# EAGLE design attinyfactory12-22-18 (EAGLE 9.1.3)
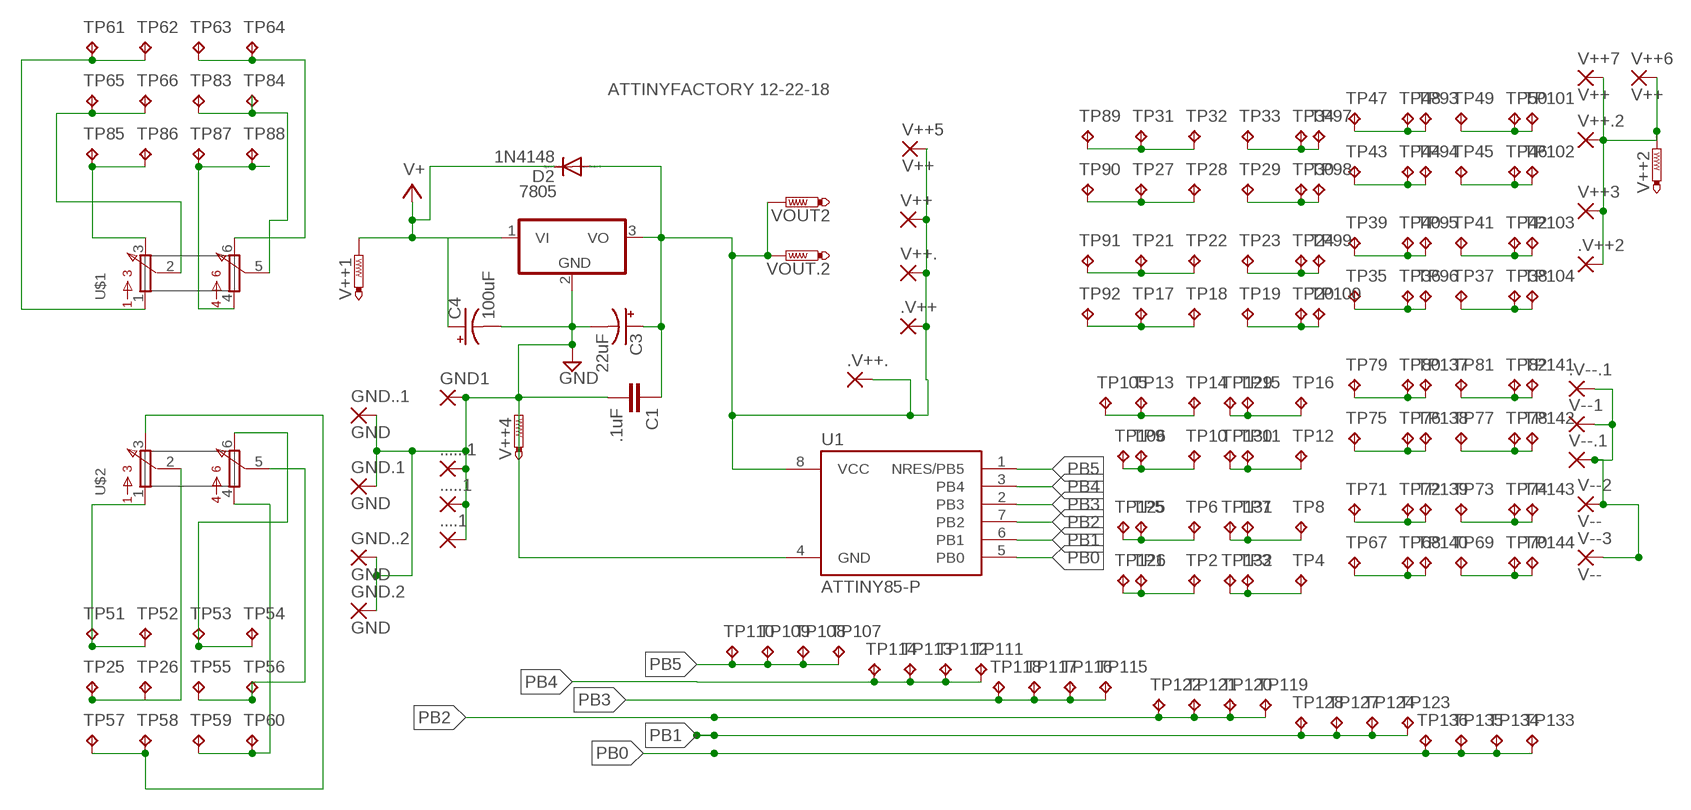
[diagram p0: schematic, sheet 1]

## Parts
7805  7805T  [TO220H]
....1  2,54/0,9  [2,54/0,9]
.....1  2,54/0,9  [2,54/0,9]
......1  2,54/0,9  [2,54/0,9]
.V++  2,54/1,0  [2,54/1,0]
.V++2  2,54/1,0  [2,54/1,0]
.V++.  2,54/1,0  [2,54/1,0]
.V--.1  3,17/1,3  [3,17/1,3]
C1  .1uF  C5/2.5  [C5B2.5]
C3  22uF  CPOL-USE3.5-10  [E3,5-10]
C4  100uF  CPOL-USE3.5-10  [E3,5-10]
D2  1N4148  1N4004  [DO41-10]
GND1  2,54/0,9  [2,54/0,9]
GND.1  GND  1,6/0,8  [1,6/0,8]
GND.2  GND  1,6/0,8  [1,6/0,8]
GND..1  GND  1,6/0,8  [1,6/0,8]
GND..2  GND  1,6/0,8  [1,6/0,8]
TP1  TPPAD1-13  [P1-13]
TP2  TPPAD1-13  [P1-13]
TP3  TPPAD1-13  [P1-13]
TP4  TPPAD1-13  [P1-13]
TP5  TPPAD1-13  [P1-13]
TP6  TPPAD1-13  [P1-13]
TP7  TPPAD1-13  [P1-13]
TP8  TPPAD1-13  [P1-13]
TP9  TPPAD1-13  [P1-13]
TP10  TPPAD1-13  [P1-13]
TP11  TPPAD1-13  [P1-13]
TP12  TPPAD1-13  [P1-13]
TP13  TPPAD1-13  [P1-13]
TP14  TPPAD1-13  [P1-13]
TP15  TPPAD1-13  [P1-13]
TP16  TPPAD1-13  [P1-13]
TP17  TPPAD1-13  [P1-13]
TP18  TPPAD1-13  [P1-13]
TP19  TPPAD1-13  [P1-13]
TP20  TPPAD1-13  [P1-13]
TP21  TPPAD1-13  [P1-13]
TP22  TPPAD1-13  [P1-13]
TP23  TPPAD1-13  [P1-13]
TP24  TPPAD1-13  [P1-13]
TP25  TPPAD1-13  [P1-13]
TP26  TPPAD1-13  [P1-13]
TP27  TPPAD1-13  [P1-13]
TP28  TPPAD1-13  [P1-13]
TP29  TPPAD1-13  [P1-13]
TP30  TPPAD1-13  [P1-13]
TP31  TPPAD1-13  [P1-13]
TP32  TPPAD1-13  [P1-13]
TP33  TPPAD1-13  [P1-13]
TP34  TPPAD1-13  [P1-13]
TP35  TPPAD1-13  [P1-13]
TP36  TPPAD1-13  [P1-13]
TP37  TPPAD1-13  [P1-13]
TP38  TPPAD1-13  [P1-13]
TP39  TPPAD1-13  [P1-13]
TP40  TPPAD1-13  [P1-13]
TP41  TPPAD1-13  [P1-13]
TP42  TPPAD1-13  [P1-13]
TP43  TPPAD1-13  [P1-13]
TP44  TPPAD1-13  [P1-13]
TP45  TPPAD1-13  [P1-13]
TP46  TPPAD1-13  [P1-13]
TP47  TPPAD1-13  [P1-13]
TP48  TPPAD1-13  [P1-13]
TP49  TPPAD1-13  [P1-13]
TP50  TPPAD1-13  [P1-13]
TP51  TPPAD1-13  [P1-13]
TP52  TPPAD1-13  [P1-13]
TP53  TPPAD1-13  [P1-13]
TP54  TPPAD1-13  [P1-13]
TP55  TPPAD1-13  [P1-13]
TP56  TPPAD1-13  [P1-13]
TP57  TPPAD1-13  [P1-13]
TP58  TPPAD1-13  [P1-13]
TP59  TPPAD1-13  [P1-13]
TP60  TPPAD1-13  [P1-13]
TP61  TPPAD1-13  [P1-13]
TP62  TPPAD1-13  [P1-13]
TP63  TPPAD1-13  [P1-13]
TP64  TPPAD1-13  [P1-13]
TP65  TPPAD1-13  [P1-13]
TP66  TPPAD1-13  [P1-13]
TP67  TPPAD1-13  [P1-13]
TP68  TPPAD1-13  [P1-13]
TP69  TPPAD1-13  [P1-13]
TP70  TPPAD1-13  [P1-13]
TP71  TPPAD1-13  [P1-13]
TP72  TPPAD1-13  [P1-13]
TP73  TPPAD1-13  [P1-13]
TP74  TPPAD1-13  [P1-13]
TP75  TPPAD1-13  [P1-13]
TP76  TPPAD1-13  [P1-13]
TP77  TPPAD1-13  [P1-13]
TP78  TPPAD1-13  [P1-13]
TP79  TPPAD1-13  [P1-13]
TP80  TPPAD1-13  [P1-13]
TP81  TPPAD1-13  [P1-13]
TP82  TPPAD1-13  [P1-13]
TP83  TPPAD1-13  [P1-13]
TP84  TPPAD1-13  [P1-13]
TP85  TPPAD1-13  [P1-13]
TP86  TPPAD1-13  [P1-13]
TP87  TPPAD1-13  [P1-13]
TP88  TPPAD1-13  [P1-13]
TP89  TPPAD1-13  [P1-13]
TP90  TPPAD1-13  [P1-13]
TP91  TPPAD1-13  [P1-13]
TP92  TPPAD1-13  [P1-13]
TP93  TPPAD1-13  [P1-13]
TP94  TPPAD1-13  [P1-13]
TP95  TPPAD1-13  [P1-13]
TP96  TPPAD1-13  [P1-13]
TP97  TPPAD1-13  [P1-13]
TP98  TPPAD1-13  [P1-13]
TP99  TPPAD1-13  [P1-13]
TP100  TPPAD1-13  [P1-13]
TP101  TPPAD1-13  [P1-13]
TP102  TPPAD1-13  [P1-13]
TP103  TPPAD1-13  [P1-13]
TP104  TPPAD1-13  [P1-13]
TP105  TPPAD1-13  [P1-13]
TP106  TPPAD1-13  [P1-13]
TP107  TPPAD1-13  [P1-13]
TP108  TPPAD1-13  [P1-13]
TP109  TPPAD1-13  [P1-13]
TP110  TPPAD1-13  [P1-13]
TP111  TPPAD1-13  [P1-13]
TP112  TPPAD1-13  [P1-13]
TP113  TPPAD1-13  [P1-13]
TP114  TPPAD1-13  [P1-13]
TP115  TPPAD1-13  [P1-13]
TP116  TPPAD1-13  [P1-13]
TP117  TPPAD1-13  [P1-13]
TP118  TPPAD1-13  [P1-13]
TP119  TPPAD1-13  [P1-13]
TP120  TPPAD1-13  [P1-13]
TP121  TPPAD1-13  [P1-13]
TP122  TPPAD1-13  [P1-13]
TP123  TPPAD1-13  [P1-13]
TP124  TPPAD1-13  [P1-13]
TP125  TPPAD1-13  [P1-13]
TP126  TPPAD1-13  [P1-13]
TP127  TPPAD1-13  [P1-13]
TP128  TPPAD1-13  [P1-13]
TP129  TPPAD1-13  [P1-13]
TP130  TPPAD1-13  [P1-13]
TP131  TPPAD1-13  [P1-13]
TP132  TPPAD1-13  [P1-13]
TP133  TPPAD1-13  [P1-13]
TP134  TPPAD1-13  [P1-13]
TP135  TPPAD1-13  [P1-13]
TP136  TPPAD1-13  [P1-13]
TP137  TPPAD1-13  [P1-13]
TP138  TPPAD1-13  [P1-13]
TP139  TPPAD1-13  [P1-13]
TP140  TPPAD1-13  [P1-13]
TP141  TPPAD1-13  [P1-13]
TP142  TPPAD1-13  [P1-13]
TP143  TPPAD1-13  [P1-13]
TP144  TPPAD1-13  [P1-13]
U1  ATTINY85-P  [PDIP08_300MIL]
U$1  DUALCONCENTRIC  [DUALCONCENTRIC]
U$2  DUALCONCENTRIC  [DUALCONCENTRIC]
V++  2,54/1,0  [2,54/1,0]
V++1  PTR1PAD1-13Y  [P1-13Y]
V++2  PTR1PAD1-13Y  [P1-13Y]
V++3  2,54/1,0  [2,54/1,0]
V++4  PTR1PAD1-13Y  [P1-13Y]
V++5  V++  1,6/0,8  [1,6/0,8]
V++6  V++  1,6/0,8  [1,6/0,8]
V++7  V++  1,6/0,8  [1,6/0,8]
V++.  2,54/1,0  [2,54/1,0]
V++.2  2,54/1,0  [2,54/1,0]
V--1  3,17/1,3  [3,17/1,3]
V--2  V--  1,6/0,8  [1,6/0,8]
V--3  V--  1,6/0,8  [1,6/0,8]
V--.1  3,17/1,3  [3,17/1,3]
VOUT2  PTR1PAD1-13Y  [P1-13Y]
VOUT.2  PTR1PAD1-13Y  [P1-13Y]

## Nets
GND: 7805.2(GND) ....1.1(P) .....1.1(P) ......1.1(P) C1.2 C3.- C4.- GND1.1(P) GND.1.1(P) GND.2.1(P) GND..1.1(P) GND..2.1(P) U1.4(GND) V++4.TP
N$1: TP1.TP TP2.TP TP126.TP
N$2: TP35.TP TP36.TP TP96.TP
N$3: TP3.TP TP4.TP TP132.TP
N$4: TP5.TP TP6.TP TP125.TP
N$5: TP7.TP TP8.TP TP131.TP
N$6: TP9.TP TP10.TP TP106.TP
N$7: TP11.TP TP12.TP TP130.TP
N$8: TP13.TP TP14.TP TP105.TP
N$9: TP15.TP TP16.TP TP129.TP
N$10: TP17.TP TP18.TP TP92.TP
N$11: TP19.TP TP20.TP TP100.TP
N$12: TP21.TP TP22.TP TP91.TP
N$13: TP23.TP TP24.TP TP99.TP
N$14: TP27.TP TP28.TP TP90.TP
N$15: TP29.TP TP30.TP TP98.TP
N$16: TP31.TP TP32.TP TP89.TP
N$17: TP33.TP TP34.TP TP97.TP
N$18: TP37.TP TP38.TP TP104.TP
N$19: TP39.TP TP40.TP TP95.TP
N$20: TP41.TP TP42.TP TP103.TP
N$21: TP43.TP TP44.TP TP94.TP
N$22: TP45.TP TP46.TP TP102.TP
N$23: TP47.TP TP48.TP TP93.TP
N$24: TP49.TP TP50.TP TP101.TP
N$25: TP51.TP TP52.TP U$2.1
N$26: .V++2.1(P) V++2.TP V++3.1(P) V++6.1(P) V++7.1(P) V++.2.1(P)
N$27: TP53.TP TP54.TP U$2.6
N$28: TP25.TP TP26.TP U$2.2
N$29: TP55.TP TP56.TP U$2.5
N$30: TP57.TP TP58.TP U$2.3
N$31: TP61.TP TP62.TP U$1.1
N$32: TP59.TP TP60.TP U$2.4
N$33: TP67.TP TP68.TP TP140.TP
N$34: TP69.TP TP70.TP TP144.TP
N$35: TP71.TP TP72.TP TP139.TP
N$36: TP63.TP TP64.TP U$1.6
N$37: TP73.TP TP74.TP TP143.TP
N$38: TP75.TP TP76.TP TP138.TP
N$39: TP77.TP TP78.TP TP142.TP
N$40: TP79.TP TP80.TP TP137.TP
N$41: TP81.TP TP82.TP TP141.TP
N$42: TP65.TP TP66.TP U$1.2
N$44: TP83.TP TP84.TP U$1.5
N$45: TP87.TP TP88.TP U$1.4
N$46: TP85.TP TP86.TP U$1.3
PB0: TP133.TP TP134.TP TP135.TP TP136.TP U1.5(PB0)
PB1: TP123.TP TP124.TP TP127.TP TP128.TP U1.6(PB1)
PB2: TP119.TP TP120.TP TP121.TP TP122.TP U1.7(PB2)
PB3: TP115.TP TP116.TP TP117.TP TP118.TP U1.2(PB3)
PB4: TP111.TP TP112.TP TP113.TP TP114.TP U1.3(PB4)
PB5: TP107.TP TP108.TP TP109.TP TP110.TP U1.1(NRES/PB5)
V+5: 7805.3(VO) .V++.1(P) .V++..1(P) C1.1 C3.+ D2.A U1.8(VCC) V++5.1(P) V++.1(P) V++..1(P) VOUT2.TP VOUT.2.TP
V+15: 7805.1(VI) C4.+ D2.C V++1.TP ; supply symbol labelled V+
V-1: .V--.1.1(P) V--1.1(P) V--2.1(P) V--3.1(P) V--.1.1(P)

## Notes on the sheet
- ATTINYFACTORY 12-22-18

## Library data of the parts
7805 = linear:78*: Positive VOLTAGE REGULATOR Source: http://cache.national.com/ds/LM/LM78L05.pdf http://www.fairchildsemi.com/ds/LM/LM7805.pdf
....1 .....1 ......1 GND1 = wirepad-NONAMES:2,54/0,9: THROUGH-HOLE PAD
.V++ .V++2 .V++. V++ V++3 V++. V++.2 = wirepad-NONAMES:2,54/1,0: THROUGH-HOLE PAD
.V--.1 V--1 V--.1 = wirepad-NONAMES:3,17/1,3: THROUGH-HOLE PAD
C1 = capacitor-wima:C: CAPACITOR
C3 C4 = rcl:CPOL-US: POLARIZED CAPACITOR, American symbol; SPICEPREFIX: C
D2 = diode:1N4004: DIODE
GND.1 GND.2 GND..1 GND..2 V++5-V++7 V--2 V--3 = wirepad-NONAMES:1,6/0,8: THROUGH-HOLE PAD
TP1-TP144 = testpad-CL:TP: Test pad NO NAME
U1 = attiny25_45_85:ATTINY85*: ATMEL ATtiny 85 Packages: P = PDIP 08 30mil S = SOIC 08 EIAJ 208mil Technologies Note: for complete ordering code (temp. range, finish, tape&reel etc.) see www.atmel.com &bull; Supply Voltage: V = (1.8&hellip;5.5)V | [blank] = (2.7&hellip;5.5)V &bull; Speed: 10 = 10 MHz | 20 = 20 MHz Author: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
U$1 U$2 = clonepots:DUALCONCENTRIC: Dual Concentric Pot Alps Clone.
V++1 V++2 V++4 VOUT2 VOUT.2 = testpad-CL:PTR1: TEST PIN

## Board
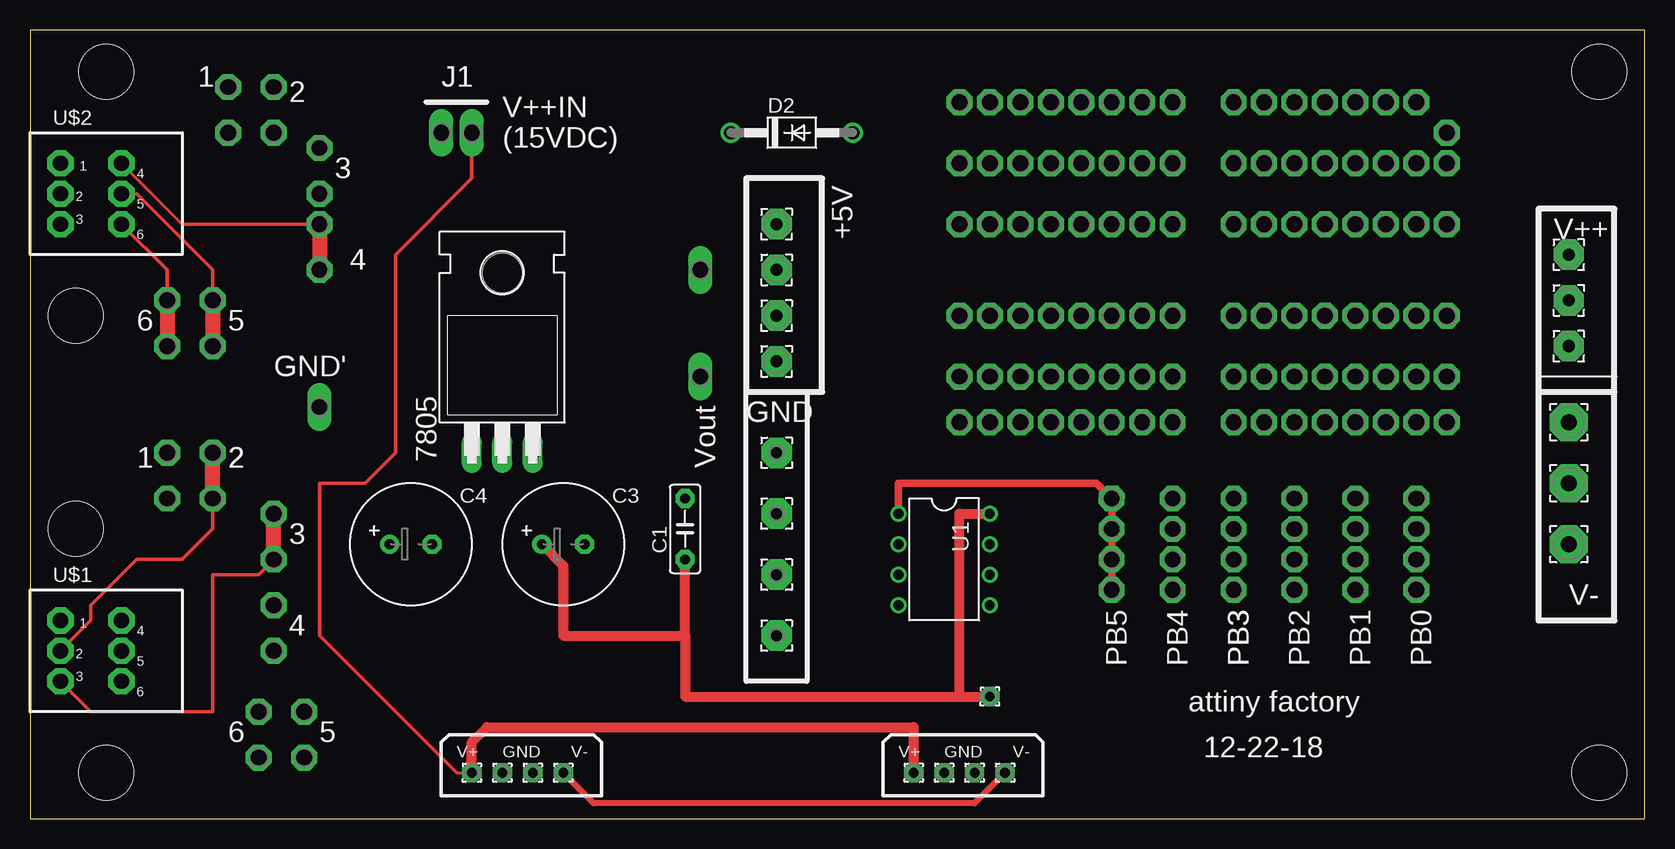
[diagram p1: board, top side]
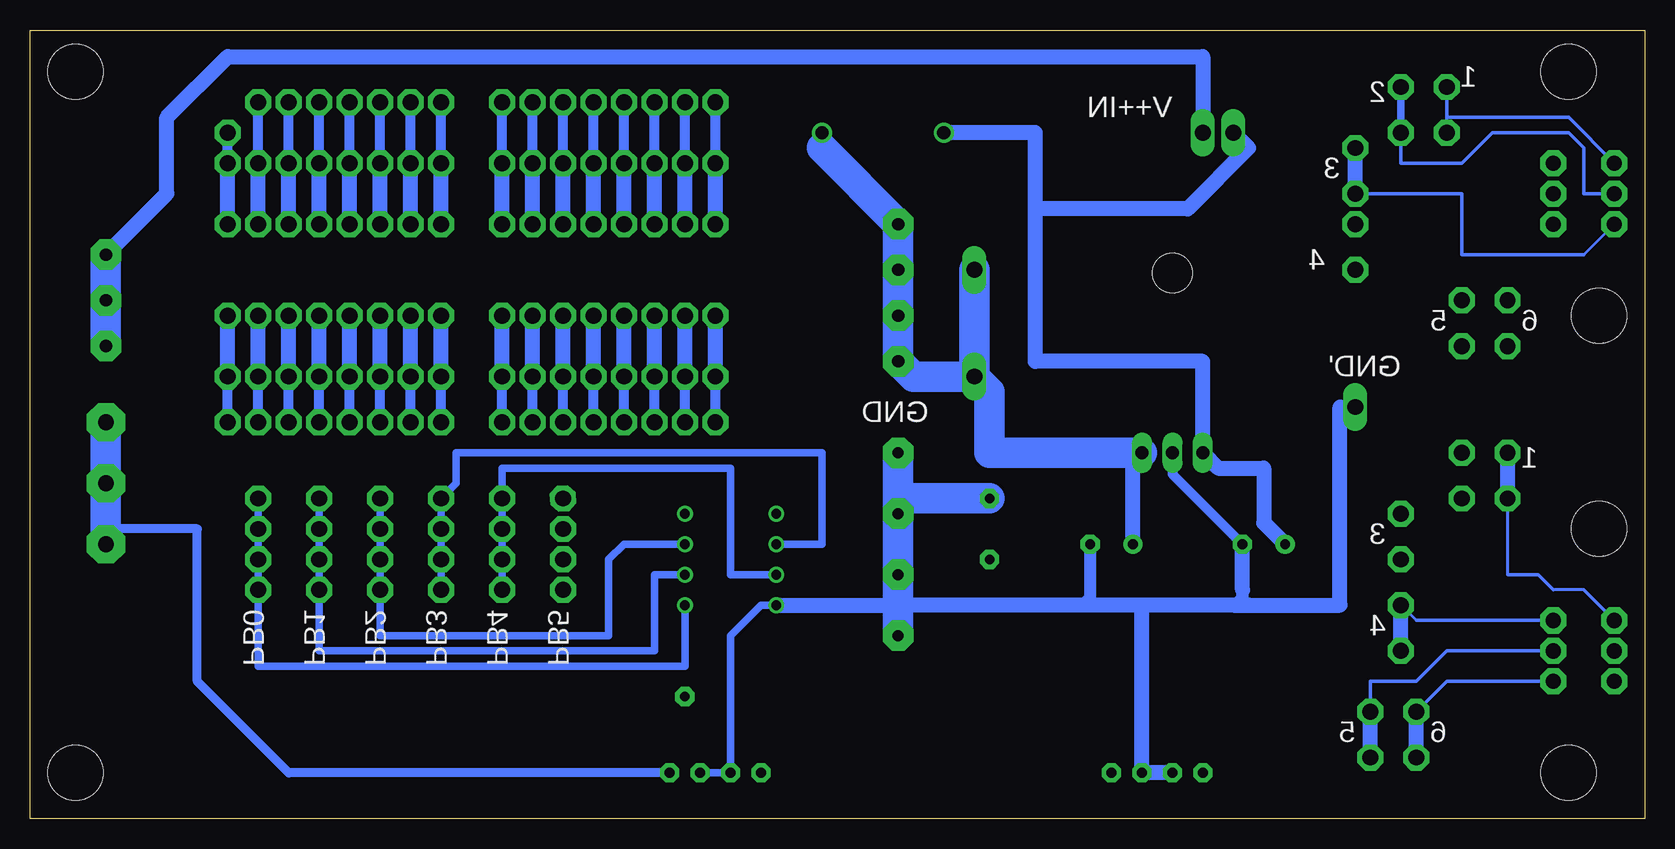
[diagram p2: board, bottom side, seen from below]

Size 134.6 x 65.71 mm. Coordinates in mm from the lower left corner, seen from the top.
Outline: 0,0 134.6,0 134.6,65.71 0,65.71 0,0
Copper layers (1*16): Top 0.035mm / dielectric 1.5mm / Bottom 0.035mm
Design rules "default": minimum track width 6mil, minimum drill 0.35mm, track to track 6mil, track to pad 6mil, pad to pad 6mil, via to via 6mil, smd to smd 6mil, copper to edge 40mil, drill to drill 6mil, minimum pad ring 10mil, minimum via ring 8mil, stop-mask expansion 4mil, vias tented up to drill 0mil, thermal gap 10mil
Holes 4.57 mm at 6.35,62.23 6.35,3.81 130.81,3.81 130.81,62.23 3.81,41.91 3.81,24.13

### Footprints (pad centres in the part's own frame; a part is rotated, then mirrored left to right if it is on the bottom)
TO220H = drill 1.118 long: 1 -2.54,-10.16; 2 0,-10.16; 3 2.54,-10.16 | hole 3.302: 0,4.826
2,54/0,9 = drill 0.914 pad 2.54 octagon: 1 0,0
2,54/1,0 = drill 1.016 pad 2.54 octagon: 1 0,0
3,17/1,3 = drill 1.321 pad 3.175 octagon: 1 0,0
C5B2.5 = drill 0.813 pad 1.6 octagon: 1 -2.54,0; 2 2.54,0
E3,5-10 = drill 0.813 pad 1.6: + -1.778,0 | drill 0.813 pad 1.6 octagon: - 1.778,0
DO41-10 = drill 1.118: A 5.08,0; C -5.08,0
1,6/0,8 = drill 0.813 pad 1.6 octagon: 1 0,0
P1-13 = drill 1.321 pad 2.159 octagon: TP 0,0
PDIP08_300MIL = drill 0.813: 1 -3.81,-3.81; 2 -1.27,-3.81; 3 1.27,-3.81; 4 3.81,-3.81; 5 3.81,3.81; 6 1.27,3.81; 7 -1.27,3.81; 8 -3.81,3.81
DUALCONCENTRIC = drill 1.27 pad 2.184 octagon: 1 -8.89,2.54; 2 -8.89,0; 3 -8.89,-2.54; 4 -3.81,2.54; 5 -3.81,0; 6 -3.81,-2.54
P1-13Y = drill 1.321 pad 1.905 long: TP 0,0

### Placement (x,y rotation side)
7805  39.37,40.64 0 top
....1  62.23,15.24 0 top
.....1  62.23,20.32 0 top
......1  62.23,25.4 0 top
.V++  62.23,45.72 0 top
.V++2  128.27,43.18 0 top
.V++.  62.23,38.1 0 top
.V--.1  128.27,22.86 0 top
C1  54.61,24.13 90 top
C3  44.45,22.86 0 top
C4  31.75,22.86 0 top
D2  63.5,57.15 0 top
GND1  62.23,30.48 0 top
GND.1  78.74,3.81 0 top
GND.2  41.91,3.81 0 top
GND..1  76.2,3.81 0 top
GND..2  39.37,3.81 0 top
TP1  95.25,36.83 0 top
TP2  95.25,41.91 0 top
TP3  92.71,36.83 0 top
TP4  92.71,41.91 0 top
TP5  90.17,36.83 0 top
TP6  90.17,41.91 0 top
TP7  87.63,36.83 0 top
TP8  87.63,41.91 0 top
TP9  85.09,36.83 0 top
TP10  85.09,41.91 0 top
TP11  82.55,36.83 0 top
TP12  82.55,41.91 0 top
TP13  80.01,36.83 0 top
TP14  80.01,41.91 0 top
TP15  77.47,36.83 0 top
TP16  77.47,41.91 0 top
TP17  95.25,49.53 0 top
TP18  95.25,54.61 0 top
TP19  92.71,49.53 0 top
TP20  92.71,54.61 0 top
TP21  90.17,49.53 0 top
TP22  90.17,54.61 0 top
TP23  87.63,49.53 0 top
TP24  87.63,54.61 0 top
TP25  20.32,60.96 0 top
TP26  20.32,57.15 0 top
TP27  85.09,49.53 0 top
TP28  85.09,54.61 0 top
TP29  82.55,49.53 0 top
TP30  82.55,54.61 0 top
TP31  80.01,49.53 0 top
TP32  80.01,54.61 0 top
TP33  77.47,49.53 0 top
TP34  77.47,54.61 0 top
TP35  118.11,49.53 0 top
TP36  118.11,54.61 0 top
TP37  115.57,49.53 0 top
TP38  115.57,54.61 0 top
TP39  113.03,49.53 0 top
TP40  113.03,54.61 0 top
TP41  110.49,49.53 0 top
TP42  110.49,54.61 0 top
TP43  107.95,49.53 0 top
TP44  107.95,54.61 0 top
TP45  105.41,49.53 0 top
TP46  105.41,54.61 0 top
TP47  102.87,49.53 0 top
TP48  102.87,54.61 0 top
TP49  100.33,49.53 0 top
TP50  100.33,54.61 0 top
TP51  16.51,57.15 0 top
TP52  16.51,60.96 0 top
TP53  11.43,39.37 0 top
TP54  11.43,43.18 0 top
TP55  15.24,43.18 0 top
TP56  15.24,39.37 0 top
TP57  24.13,55.88 0 top
TP58  24.13,52.07 0 top
TP59  24.13,49.53 0 top
TP60  24.13,45.72 0 top
TP61  11.43,30.48 0 top
TP62  11.43,26.67 0 top
TP63  19.05,8.89 0 top
TP64  19.05,5.08 0 top
TP65  15.24,26.67 0 top
TP66  15.24,30.48 0 top
TP67  118.11,36.83 0 top
TP68  118.11,41.91 0 top
TP69  115.57,36.83 0 top
TP70  115.57,41.91 0 top
TP71  113.03,36.83 0 top
TP72  113.03,41.91 0 top
TP73  110.49,36.83 0 top
TP74  110.49,41.91 0 top
TP75  107.95,36.83 0 top
TP76  107.95,41.91 0 top
TP77  105.41,36.83 0 top
TP78  105.41,41.91 0 top
TP79  102.87,36.83 0 top
TP80  102.87,41.91 0 top
TP81  100.33,36.83 0 top
TP82  100.33,41.91 0 top
TP83  22.86,5.08 0 top
TP84  22.86,8.89 0 top
TP85  20.32,25.4 0 top
TP86  20.32,21.59 0 top
TP87  20.32,13.97 0 top
TP88  20.32,17.78 0 top
TP89  80.01,59.69 0 top
TP90  85.09,59.69 0 top
TP91  90.17,59.69 0 top
TP92  95.25,59.69 0 top
TP93  102.87,59.69 0 top
TP94  107.95,59.69 0 top
TP95  113.03,59.69 0 top
TP96  118.11,57.15 0 top
TP97  77.47,59.69 0 top
TP98  82.55,59.69 0 top
TP99  87.63,59.69 0 top
TP100  92.71,59.69 0 top
TP101  100.33,59.69 0 top
TP102  105.41,59.69 0 top
TP103  110.49,59.69 0 top
TP104  115.57,59.69 0 top
TP105  80.01,33.02 0 top
TP106  85.09,33.02 0 top
TP107  90.17,26.67 356.7 top
TP108  90.17,24.13 0 top
TP109  90.17,21.59 0 top
TP110  90.17,19.05 0 top
TP111  95.25,26.67 0 top
TP112  95.25,24.13 180 top
TP113  95.25,21.59 0 top
TP114  95.25,19.05 0 top
TP115  100.33,26.67 0 top
TP116  100.33,24.13 180 top
TP117  100.33,21.59 0 top
TP118  100.33,19.05 0 top
TP119  105.41,24.13 0 top
TP120  105.41,21.59 0 top
TP121  105.41,19.05 0 top
TP122  105.41,26.67 0 top
TP123  110.49,21.59 0 top
TP124  110.49,19.05 0 top
TP125  90.17,33.02 0 top
TP126  95.25,33.02 0 top
TP127  110.49,26.67 0 top
TP128  110.49,24.13 0 top
TP129  77.47,33.02 0 top
TP130  82.55,33.02 0 top
TP131  87.63,33.02 0 top
TP132  92.71,33.02 0 top
TP133  115.57,19.05 0 top
TP134  115.57,26.67 0 top
TP135  115.57,24.13 0 top
TP136  115.57,21.59 0 top
TP137  102.87,33.02 0 top
TP138  107.95,33.02 0 top
TP139  113.03,33.02 0 top
TP140  118.11,33.02 0 top
TP141  100.33,33.02 0 top
TP142  105.41,33.02 0 top
TP143  110.49,33.02 0 top
TP144  115.57,33.02 0 top
U1  76.2,21.59 270 top
U$1  11.43,13.97 0 top
U$2  11.43,52.07 0 top
V++  62.23,41.91 0 top
V++1  34.29,57.15 0 top
V++2  36.83,57.15 0 top
V++3  128.27,46.99 0 top
V++4  24.13,34.29 0 top
V++5  80.01,10.16 0 top
V++6  73.66,3.81 0 top
V++7  36.83,3.81 0 top
V++.  62.23,49.53 0 top
V++.2  128.27,39.37 0 top
V--1  128.27,27.94 0 top
V--2  81.28,3.81 0 top
V--3  44.45,3.81 0 top
V--.1  128.27,33.02 0 top
VOUT2  55.88,45.72 0 top
VOUT.2  55.88,36.83 0 top

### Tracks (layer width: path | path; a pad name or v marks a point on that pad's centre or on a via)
GND
  Bottom 0.61: U1.4 73.66,17.78 76.2,15.24 GND..1.1 GND.1.1
  Bottom 0.813: 46.23,18.54 46.99,17.78 | 33.53,18.54 34.29,17.78 | 7805.2 39.37,28.7 C4.-
  Bottom 1.016: C3.- 46.23,20.32 46.23,18.54 | 33.53,18.54 33.53,19.05
  Bottom 1.27: 33.02,17.78 34.29,17.78 | 34.29,17.78 41.91,17.78 | 41.91,17.78 43.18,17.78 46.99,17.78 62.23,17.78 U1.4 | GND..2.1 GND.2.1 41.91,17.78 | 33.53,19.05 C4.- | 34.29,17.78 25.4,17.78 25.4,34.29 V++4.TP
  Bottom 2.54: ....1.1 62.23,17.78 .....1.1 ......1.1 62.23,26.67 | 62.23,26.67 GND1.1 | C1.2 62.23,26.67
N$1
  Bottom 0.813: TP126.TP TP1.TP
  Bottom 1.27: TP1.TP TP2.TP
N$2
  Bottom 0.813: TP36.TP TP96.TP
  Bottom 1.27: TP35.TP TP36.TP
N$3
  Bottom 0.813: TP132.TP TP3.TP
  Bottom 1.27: TP3.TP TP4.TP
N$4
  Bottom 0.813: TP125.TP TP5.TP
  Bottom 1.27: TP5.TP TP6.TP
N$5
  Bottom 0.813: TP131.TP TP7.TP
  Bottom 1.27: TP7.TP TP8.TP
N$6
  Bottom 0.813: TP106.TP TP9.TP
  Bottom 1.27: TP9.TP TP10.TP
N$7
  Bottom 0.813: TP130.TP TP11.TP
  Bottom 1.27: TP11.TP TP12.TP
N$8
  Bottom 0.813: TP105.TP TP13.TP
  Bottom 1.27: TP13.TP TP14.TP
N$9
  Bottom 0.813: TP129.TP TP15.TP
  Bottom 1.27: TP15.TP TP16.TP
N$10
  Bottom 0.813: TP18.TP TP92.TP
  Bottom 1.27: TP17.TP TP18.TP
N$11
  Bottom 0.813: TP20.TP TP100.TP
  Bottom 1.27: TP19.TP TP20.TP
N$12
  Bottom 0.813: TP22.TP TP91.TP
  Bottom 1.27: TP21.TP TP22.TP
N$13
  Bottom 0.813: TP24.TP TP99.TP
  Bottom 1.27: TP23.TP TP24.TP
N$14
  Bottom 0.813: TP28.TP TP90.TP
  Bottom 1.27: TP27.TP TP28.TP
N$15
  Bottom 0.813: TP30.TP TP98.TP
  Bottom 1.27: TP29.TP TP30.TP
N$16
  Bottom 0.813: TP32.TP TP89.TP
  Bottom 1.27: TP31.TP TP32.TP
N$17
  Bottom 0.813: TP34.TP TP97.TP
  Bottom 1.27: TP33.TP TP34.TP
N$18
  Bottom 0.813: TP38.TP TP104.TP
  Bottom 1.27: TP37.TP TP38.TP
N$19
  Bottom 0.813: TP40.TP TP95.TP
  Bottom 1.27: TP39.TP TP40.TP
N$20
  Bottom 0.813: TP42.TP TP103.TP
  Bottom 1.27: TP41.TP TP42.TP
N$21
  Bottom 0.813: TP44.TP TP94.TP
  Bottom 1.27: TP43.TP TP44.TP
N$22
  Bottom 0.813: TP46.TP TP102.TP
  Bottom 1.27: TP45.TP TP46.TP
N$23
  Bottom 0.813: TP48.TP TP93.TP
  Bottom 1.27: TP47.TP TP48.TP
N$24
  Bottom 0.813: TP50.TP TP101.TP
  Bottom 1.27: TP49.TP TP50.TP
N$25
  Bottom 0.254: 16.51,58.42 TP51.TP
  Bottom 0.305: U$2.1 6.35,58.42 16.51,58.42 | TP51.TP TP52.TP
N$26
  Top 0.254: 35.56,3.81 V++7.1
  Top 0.305: 35.56,3.81 24.13,15.24 24.13,27.94 27.94,27.94 30.48,30.48 30.48,46.99 36.83,53.34 V++2.TP
  Top 0.813: V++7.1 36.83,6.35 38.1,7.62 73.66,7.62 V++6.1
  Bottom 1.27: V++3.1 123.19,52.07 123.19,58.42 118.11,63.5 36.83,63.5 V++2.TP
  Bottom 2.54: V++3.1 .V++2.1 V++.2.1
N$27
  Top 0.305: U$2.6 11.43,45.72 TP54.TP
  Top 1.27: TP54.TP TP53.TP
N$28
  Bottom 0.305: U$2.2 5.08,52.07 5.08,55.88 6.35,57.15 12.7,57.15 15.24,54.61 20.32,54.61 TP26.TP
  Bottom 0.61: TP25.TP TP26.TP
N$29
  Top 0.254: U$2.5 8.89,52.07
  Top 0.305: 8.89,52.07 15.24,45.72 TP55.TP
  Top 1.27: TP55.TP TP56.TP
N$30
  Bottom 0.254: U$2.3 5.08,46.99
  Bottom 0.305: 5.08,46.99 15.24,46.99 15.24,52.07 TP58.TP
  Bottom 1.27: TP58.TP TP57.TP
N$31
  Bottom 0.254: 5.08,19.05 7.62,19.05 | 11.43,20.32 TP62.TP
  Bottom 0.305: U$1.1 5.08,19.05 | 7.62,19.05 8.89,20.32 11.43,20.32
  Bottom 1.27: TP62.TP TP61.TP
N$32
  Top 0.254: U$2.4 12.7,49.53
  Top 0.305: 12.7,49.53 TP59.TP
  Top 1.27: TP59.TP TP60.TP
N$33
  Bottom 0.813: TP140.TP TP67.TP
  Bottom 1.27: TP67.TP TP68.TP
N$34
  Bottom 0.813: TP144.TP TP69.TP
  Bottom 1.27: TP69.TP TP70.TP
N$35
  Bottom 0.813: TP139.TP TP71.TP
  Bottom 1.27: TP71.TP TP72.TP
N$36
  Bottom 0.305: U$1.6 16.51,11.43 TP63.TP
  Bottom 1.27: TP64.TP TP63.TP
N$37
  Bottom 0.813: TP143.TP TP73.TP
  Bottom 1.27: TP73.TP TP74.TP
N$38
  Bottom 0.813: TP138.TP TP75.TP
  Bottom 1.27: TP75.TP TP76.TP
N$39
  Bottom 0.813: TP142.TP TP77.TP
  Bottom 1.27: TP77.TP TP78.TP
N$40
  Bottom 0.813: TP137.TP TP79.TP
  Bottom 1.27: TP79.TP TP80.TP
N$41
  Bottom 0.813: TP141.TP TP81.TP
  Bottom 1.27: TP81.TP TP82.TP
N$42
  Top 0.305: U$1.2 5.08,16.51 5.08,17.78 8.89,21.59 12.7,21.59 15.24,24.13 TP65.TP
  Top 1.27: TP65.TP TP66.TP
N$44
  Bottom 0.305: U$1.5 16.51,13.97 19.05,11.43 22.86,11.43 TP84.TP
  Bottom 1.27: TP83.TP TP84.TP
N$45
  Bottom 0.254: 19.05,16.51 TP88.TP
  Bottom 0.305: U$1.4 19.05,16.51
  Bottom 1.27: TP87.TP TP88.TP
N$46
  Top 0.305: U$1.3 5.08,8.89 15.24,8.89 15.24,20.32 19.05,20.32 TP86.TP
  Top 1.27: TP86.TP TP85.TP
PB0
  Bottom 0.61: TP134.TP TP135.TP TP136.TP TP133.TP 115.57,12.7 80.01,12.7 U1.5
PB1
  Bottom 0.61: TP127.TP TP128.TP TP123.TP TP124.TP 110.49,13.97 82.55,13.97 82.55,20.32 U1.6
PB2
  Bottom 0.61: U1.7 85.09,22.86 86.36,21.59 86.36,15.24 105.41,15.24 TP121.TP TP120.TP TP119.TP TP122.TP
PB3
  Bottom 0.61: TP118.TP TP117.TP TP116.TP TP115.TP 99.06,27.94 99.06,30.48 68.58,30.48 68.58,22.86 U1.2
PB4
  Bottom 0.61: TP114.TP TP113.TP TP112.TP TP111.TP 95.25,29.21 76.2,29.21 76.2,20.32 U1.3
PB5
  Top 0.61: U1.1 72.39,27.94 88.9,27.94 TP107.TP TP108.TP TP109.TP TP110.TP
V+5
  Top 0.813: C3.+ 44.45,21.08 44.45,15.24 54.61,15.24 | 54.61,15.24 C1.1 | 54.61,15.24 54.61,10.16 77.47,10.16 | 77.47,10.16 77.47,25.4 U1.8 | 77.47,10.16 V++5.1
  Bottom 1.27: 68.58,55.88 D2.A | C3.+ 42.67,29.72 7805.3
  Bottom 2.54: 68.58,55.88 V++..1 .V++.1 V++.1 .V++..1 60.96,36.83 VOUT.2.TP | VOUT.2.TP VOUT2.TP | VOUT.2.TP 54.61,35.56 54.61,30.48 7805.3
V+15
  Bottom 1.27: 50.8,50.8 50.8,38.1 36.83,38.1 7805.1 35.56,29.21 31.75,29.21 31.75,24.64 C4.+ | 50.8,50.8 50.8,57.15 D2.C | V++1.TP 33.02,55.88 38.1,50.8 50.8,50.8
V-1
  Top 0.508: V--2.1 78.74,1.27 46.99,1.27 V--3.1
  Bottom 0.61: 127,24.13 .V--.1.1
  Bottom 0.762: V--2.1 113.03,3.81 120.65,11.43 120.65,24.13 127,24.13
  Bottom 2.54: V--.1.1 V--1.1 .V--.1.1

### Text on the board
tNames: 1 | J1 | 2 | V++IN | (15VDC) | 3 | +5V | V++ | 4 | 6 | 5 | GND' | GND | 1 | 2 | 2 | Vout | 3 | V- | 4 | PB5 | PB4 | PB3 | PB3 | PB2 | PB1 | PB0 | attiny factory | 6 | 5 | V+ | GND | V- | V+ | GND | V- | 12-22-18
bNames: 1 | 2 | V++IN | 3 | 4 | 6 | 5 | GND' | GND | 1 | 3 | 4 | PB5 | PB4 | PB3 | PB2 | PB1 | PB0 | 6 | 5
